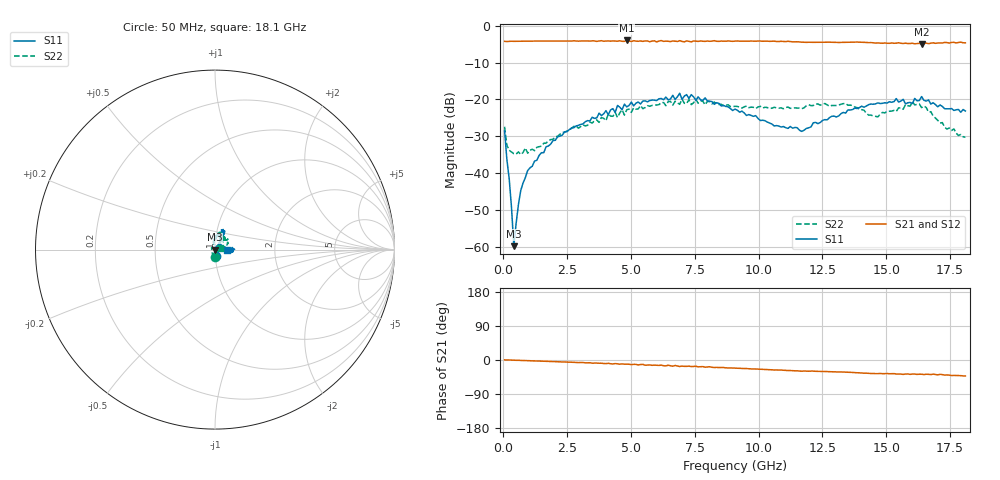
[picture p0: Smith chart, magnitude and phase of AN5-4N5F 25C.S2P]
! Network Analyzer HP8720D.06.14 Serial No. US36140669
! 28 Jun 2005  12:38:12
! Frequency  S11  S21  S12  S22
# HZ  S  DB R 50
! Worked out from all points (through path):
!   201 points, 50 MHz to 18.1 GHz, reference 50 ohm
!   highest |S21| = -4.01 dB at 4.833 GHz (marker M1); lowest = -4.9 dB at 16.39 GHz (marker M2)
!   group delay of S21, straight-line fit = 6.64 ps
!   lowest |S11| = -59.8 dB at 411 MHz (marker M3), VSWR 1.00, Z = 49.9 - j0.0204 ohm
!   |S11| at or under -10 dB: start of sweep to end of sweep
!   |S22| runs from -35.0 to -19.9 dB; largest |S21 - S12| = 0.021
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5e7  -28.58 -85.7  -4.26 0.4  -4.25 0.5  -27.43 -91.4
1.4025e8  -36.40 -93.7  -4.30 0.0  -4.27 0.0  -32.44 -140.0
3.2075e8  -49.36 -112.0  -4.22 -0.2  -4.25 -0.2  -34.26 -171.5
4.11e8  -59.81 -168.4  -4.25 -0.6  -4.24 -0.6  -34.72 -179.7
6.8175e8  -44.73 81.0  -4.22 -1.1  -4.22 -1.1  -34.96 159.3
9.525e8  -39.32 67.1  -4.20 -1.6  -4.20 -1.7  -34.58 145.6
1.94525e9  -31.15 58.5  -4.17 -4.1  -4.18 -4.2  -30.82 109.5
3.1185e9  -26.66 58.5  -4.15 -6.6  -4.18 -7.0  -26.90 101.6
4.83325e9  -22.02 64.0  -4.01 -11.1  -4.13 -11.6  -22.79 81.3
6.09675e9  -19.83 61.9  -4.18 -14.3  -4.09 -14.3  -21.42 78.1
6.909e9  -18.34 68.0  -4.07 -17.1  -4.15 -16.1  -21.34 70.2
6.99925e9  -19.97 67.3  -4.27 -16.0  -4.37 -17.3  -19.88 71.7
7.36025e9  -18.70 61.5  -4.40 -17.3  -4.21 -16.8  -21.42 75.9
9.075e9  -22.63 67.7  -4.18 -21.5  -4.16 -21.6  -21.86 57.8
1.169225e10  -28.68 19.5  -4.47 -29.5  -4.47 -29.5  -22.52 56.2
1.21435e10  -26.33 20.9  -4.51 -29.3  -4.47 -29.6  -21.65 54.5
1.3407e10  -23.71 4.1  -4.48 -31.9  -4.46 -32.3  -21.11 51.1
1.46705e10  -20.95 -11.7  -4.68 -36.0  -4.67 -36.0  -24.73 54.0
1.512175e10  -20.64 -7.7  -4.79 -36.3  -4.66 -36.4  -23.22 53.3
1.602425e10  -21.12 1.0  -4.77 -37.2  -4.93 -38.6  -20.63 39.0
1.638525e10  -19.22 0.5  -4.94 -37.6  -4.75 -37.7  -22.22 28.3
1.81e10  -23.15 -0.4  -4.66 -42.1  -4.70 -42.7  -30.27 13.5
